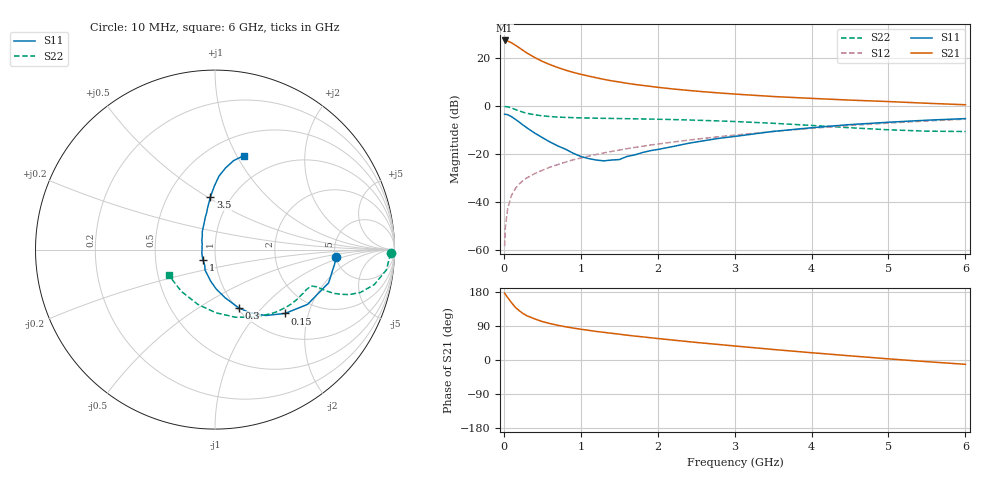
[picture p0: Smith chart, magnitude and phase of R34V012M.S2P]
! SIEMENS Small Signal Semiconductors
! BFR181
! Si NPN RF Bipolar Junction Transistor in SOT23
! VCE = 4 V  IC = 12 mA
! Common Emitter S-Parameters:  May  1996
# GHz  S  MA  R  50
!  f  S11  S21  S12  S22
! GHz  MAG  ANG  MAG  ANG  MAG  ANG  MAG  ANG
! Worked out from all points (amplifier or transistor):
!   36 points, 10 MHz to 6 GHz, reference 50 ohm
!   highest |S21| = 27.3 dB at 10 MHz (marker M1)
!   |S21| within 3 dB of that: start of sweep to 197.6 MHz
!   unconditionally stable (mu >= 1): 700.8 MHz to 2.613 GHz
!   at 250 MHz: K = 0.65, MSG = 27.1 dB, |S12| = -31.0 dB
!   at 1.4 GHz: K = 1.06, MAG = 13.2 dB, |S12| = -18.9 dB
!   at 6 GHz: K = 0.85, MSG = 3.0 dB, |S12| = -5.5 dB
!   S11 on the Smith chart (normalised r, x): 10 MHz: 5.05, -0.72; 150 MHz: 1.45, -1.43; 300 MHz: 1.02, -0.76; 1 GHz: 0.87, -0.10; 3.5 GHz: 0.80, +0.52; 6 GHz: 0.72, +1.07
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0.01  0.6751 -3.3  23.24 176.4  0.0012 81.7  0.9801 -1.2
0.02  0.6722 -6.4  22.96 173.3  0.003 87.7  0.9728 -2.8
0.05  0.6596 -16.3  22.53 164.7  0.0073 83.9  0.9614 -6.8
0.1  0.5993 -30.6  20.8 151.1  0.0138 77.1  0.9085 -12.4
0.15  0.5278 -42.4  18.48 139.0  0.0191 72.9  0.8449 -16.4
0.2  0.4628 -52.5  16.36 130.1  0.0238 70.9  0.7897 -18.5
0.25  0.4005 -61.3  14.42 122.6  0.0281 69.6  0.7422 -19.6
0.3  0.3514 -67.7  12.74 116.7  0.0318 69.2  0.7058 -20.2
0.4  0.2739 -78.2  10.29 108.6  0.039 69.4  0.6568 -20.4
0.5  0.2199 -88.2  8.511 101.4  0.0458 70.5  0.6243 -20.2
0.6  0.1781 -97.7  7.286 96.2  0.0532 70.8  0.6026 -20.1
0.7  0.1478 -106.2  6.354 91.7  0.06 71.3  0.5886 -20.4
0.8  0.1264 -116.1  5.613 87.8  0.0676 71.2  0.5795 -20.5
1  0.0889 -138.7  4.584 81.2  0.0823 71.5  0.5662 -21.7
1.1  0.0803 -152.2  4.212 78.4  0.0901 71.1  0.5619 -22.6
1.3  0.0719 179.9  3.593 73.0  0.1056 70.7  0.554 -24.2
1.6  0.0887 145.8  2.976 65.5  0.1289 69.6  0.5446 -27.4
2.2  0.1433 116.9  2.265 52.6  0.1779 66.2  0.522 -35.4
3.5  0.2954 94.9  1.578 27.8  0.2943 55.4  0.4368 -59.4
4.5  0.4102 86.9  1.328 11.0  0.3929 44.3  0.3522 -89.1
5.5  0.5064 78.2  1.142 -4.4  0.4883 31.3  0.299 -128.9
6  0.5464 73.1  1.062 -11.4  0.5315 24.2  0.2941 -151.0
